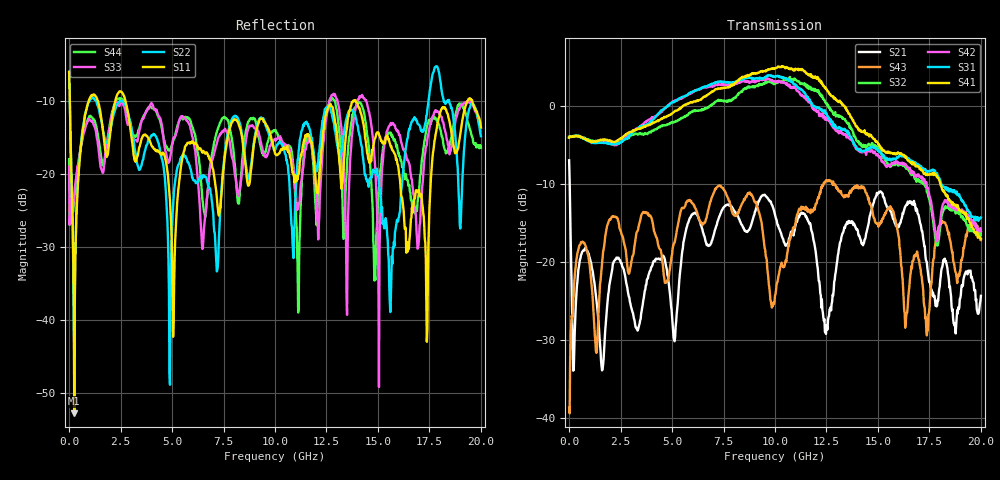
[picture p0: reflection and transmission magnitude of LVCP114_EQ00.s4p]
!Agilent Technologies,N5230A,MY46400459,A.07.50.48
!Agilent N5230A: A.07.50.48
!Date: Monday, January 09, 2012 13:59:45
!Correction: S11(Full 4 Port(1,2,3,4))
!S12(Full 4 Port(1,2,3,4))
!S13(Full 4 Port(1,2,3,4))
!S14(Full 4 Port(1,2,3,4))
!S21(Full 4 Port(1,2,3,4))
!S22(Full 4 Port(1,2,3,4))
!S23(Full 4 Port(1,2,3,4))
!S24(Full 4 Port(1,2,3,4))
!S31(Full 4 Port(1,2,3,4))
!S32(Full 4 Port(1,2,3,4))
!S33(Full 4 Port(1,2,3,4))
!S34(Full 4 Port(1,2,3,4))
!S41(Full 4 Port(1,2,3,4))
!S42(Full 4 Port(1,2,3,4))
!S43(Full 4 Port(1,2,3,4))
!S44(Full 4 Port(1,2,3,4))
!S4P File: Measurements: <S11,S12,S13,S14>,
!<S21,S22,S23,S24>,
!<S31,S32,S33,S34>,
!<S41,S42,S43,S44>:
# Hz S  dB  R 50
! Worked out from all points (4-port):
!   801 points, 300 kHz to 20 GHz, reference 50 ohm
!   strongest paths, dB at 300 kHz, 5 GHz, 10 GHz, 15 GHz, 20 GHz:
!     S41: -4.1, -1.0, 4.8, -4.8, -17.1
!     S31: -4.1, 0.4, 3.7, -5.8, -14.4
!     S42: -4.1, 0.4, 3.1, -6.3, -16.1
!     S32: -4.0, -2.2, 2.8, -5.6, -16.2
!     S43: -38.7, -19.1, -24.3, -15.1, -17.2
!     S21: -7.0, -27.1, -14.0, -11.3, -24.4
!   lowest |S11| = -52.8 dB at 250.3 MHz (marker M1), VSWR 1.00, Z = 50.2 + j0.0408 ohm
!   |S11| at or under -10 dB: 34.61 MHz to 949.8 MHz (915.2 MHz wide, 186 % of centre); 2.737 GHz to 13.79 GHz (11.06 GHz wide, 134 % of centre); 13.91 GHz to 19.35 GHz (5.436 GHz wide, 32.7 % of centre)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
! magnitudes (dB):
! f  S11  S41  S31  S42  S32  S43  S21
! 300 kHz  -6.0  -4.1  -4.1  -4.1  -4.0  -38.7  -7.0
! 250.3 MHz  -52.8  -4.0  -4.0  -3.9  -3.9  -22.7  -31.2
! 1.15 GHz  -9.1  -4.6  -4.7  -4.7  -4.5  -24.9  -21.3
! 4.9 GHz  -23.7  -1.2  0.2  0.2  -2.2  -20.8  -24.2
! 8.025 GHz  -12.5  2.8  3.0  2.8  0.9  -14.1  -13.6
! 15.6 GHz  -16.0  -6.1  -7.0  -7.7  -7.9  -12.9  -13.5
! 20 GHz  -13.6  -17.1  -14.4  -16.1  -16.2  -17.2  -24.4
